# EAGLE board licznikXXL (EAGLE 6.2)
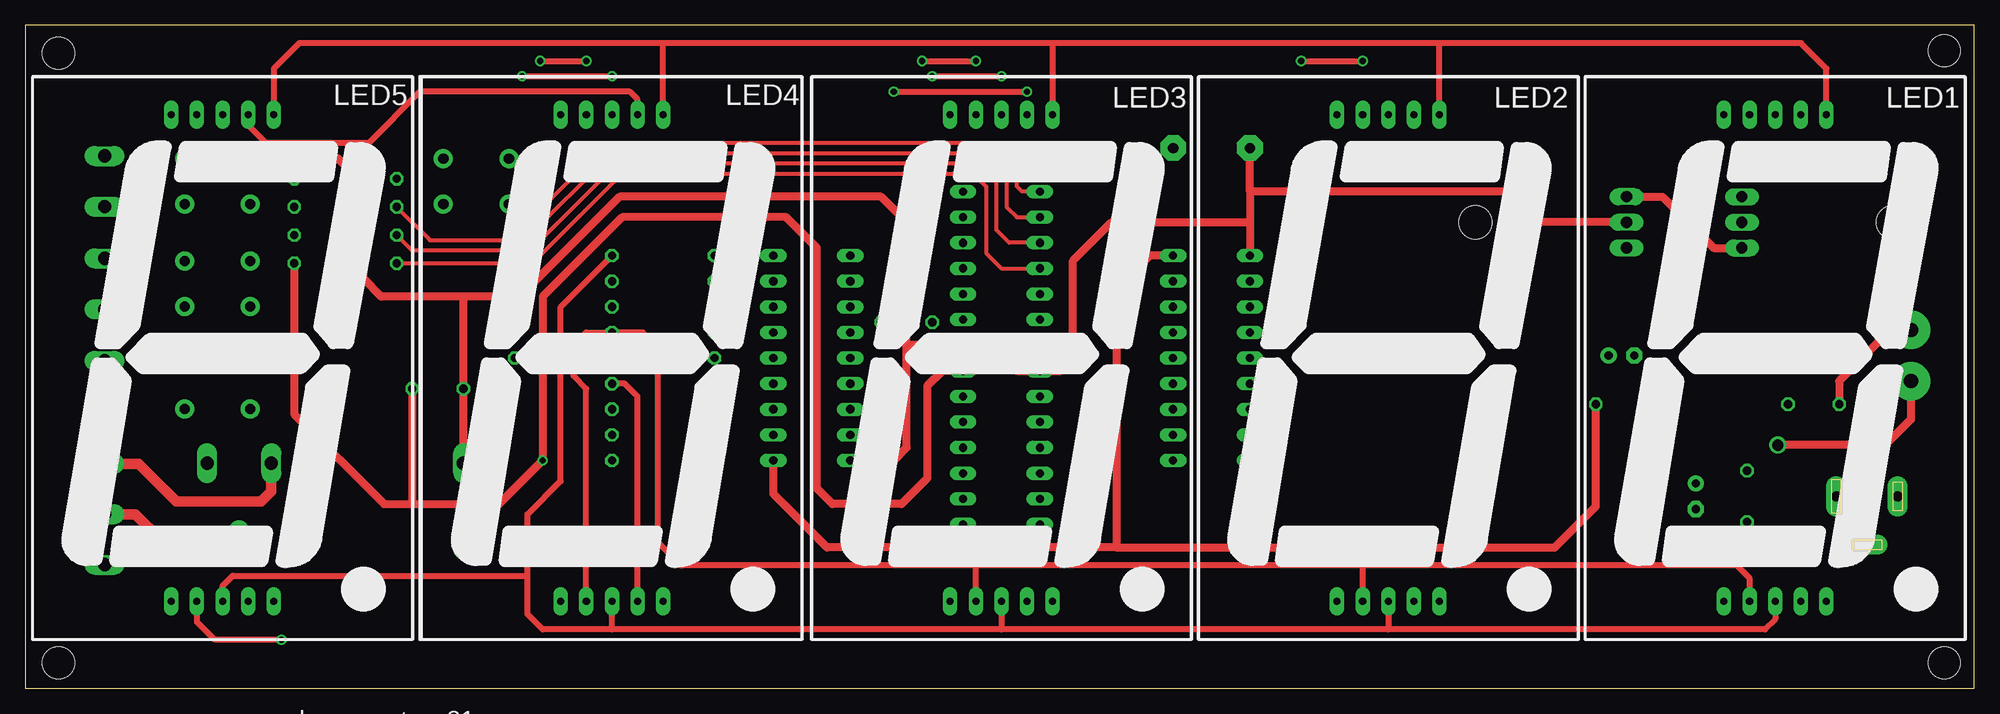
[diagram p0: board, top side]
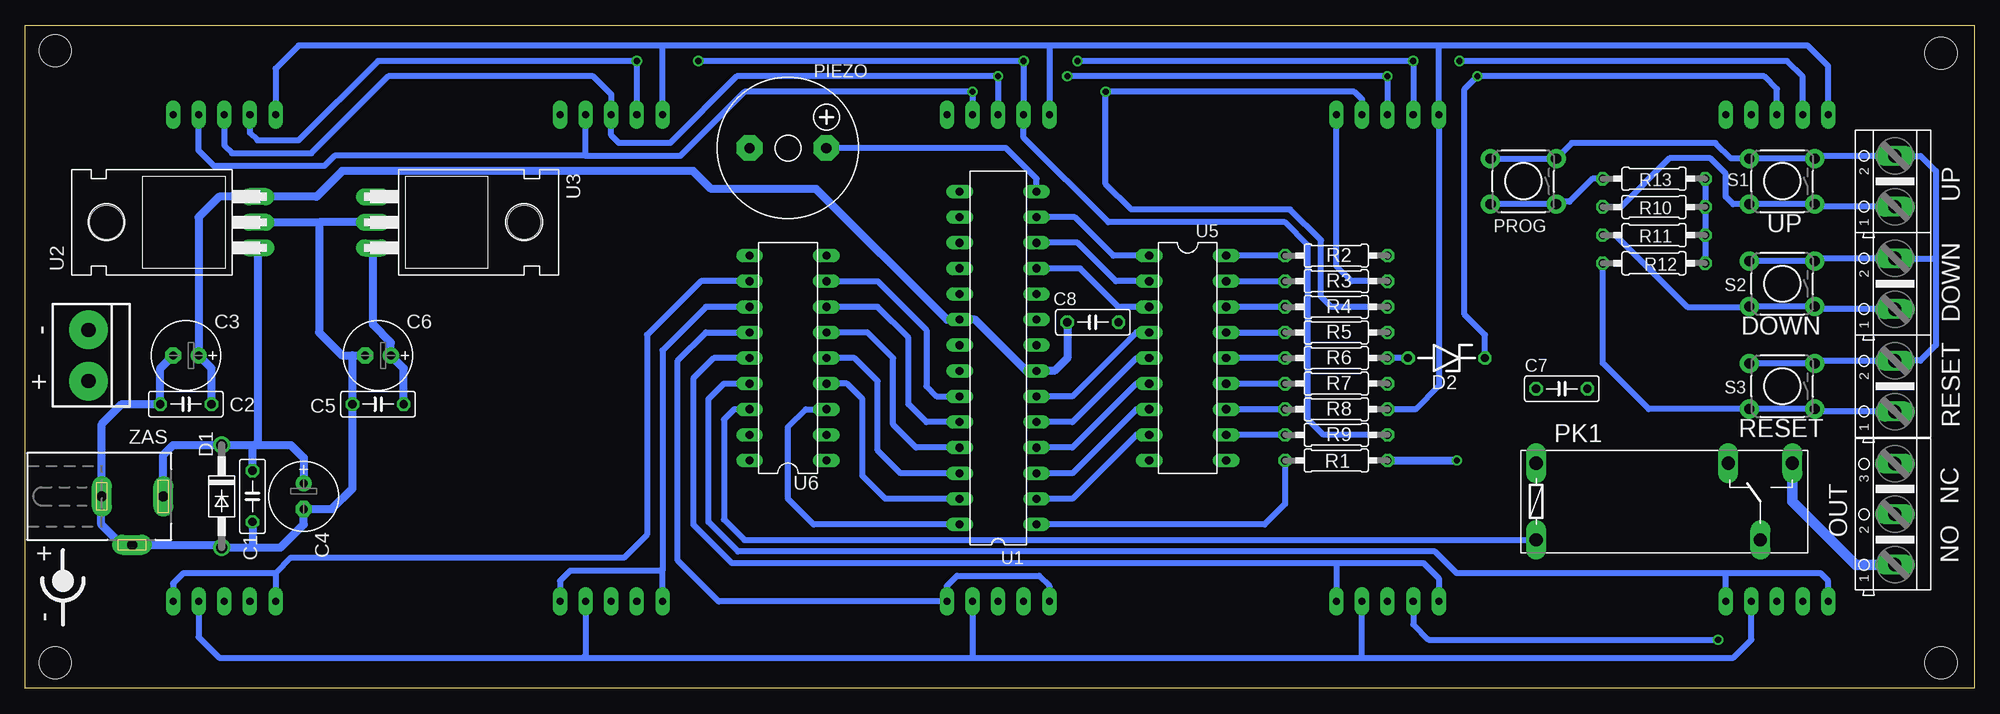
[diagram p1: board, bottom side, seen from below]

Size 193.22 x 65.78 mm. Coordinates in mm from the lower left corner, seen from the top.
Outline: 0,0 193.22,0 193.22,65.78 0,65.78 0,0
Copper layers (1*16): Top 0.035mm / dielectric 1.5mm / Bottom 0.035mm
Design rules: minimum track width 10mil, minimum drill 24mil, track to track 8mil, track to pad 8mil, pad to pad 8mil, via to via 8mil, smd to smd 8mil, copper to edge 40mil, drill to drill 8mil, minimum pad ring 10mil, minimum via ring 8mil, stop-mask expansion 4mil, vias tented up to drill 0mil, thermal gap 10mil
Holes 3.2 mm at 3.3,62.99 3.3,2.54 190.25,2.54 190.25,63.25

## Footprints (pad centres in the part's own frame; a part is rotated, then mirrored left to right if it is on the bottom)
C050-025X075 = drill 0.813 octagon: 1 -2.54,0; 2 2.54,0
E2,5-7 = drill 0.813 pad 1.6: + -1.27,0 | drill 0.813 pad 1.6 octagon: - 1.27,0
DO41-10 = drill 1.118: A 5.08,0; C -5.08,0
ZDIO-7.5 = drill 0.813 octagon: A 3.81,0; C -3.81,0
AK500/2 = drill 1.321 long: 1 -2.515,0; 2 2.515,0
SA18-11 = drill 0.7 pad 1.422 long: 1 -5.08,-24.13; 2 -2.54,-24.13; 3 0,-24.13; 4 2.54,-24.13; 5 5.08,-24.13; 6 -5.08,24.13; 7 -2.54,24.13; 8 0,24.13; 9 2.54,24.13; 10 5.08,24.13
AK500/3 = drill 1.321 long: 1 -5.004,0; 2 0,0; 3 5.004,0
F/CM12P = drill 1.016 pad 2.54 octagon: + 3.81,0; - -3.81,0
G6RW = drill 1.321 long: 1 -12.7,-3.81; 2 -12.7,3.81; O 6.35,3.81; P 9.525,-3.81; S 12.7,3.81
TACTILE-PTH = drill 1.016 pad 1.88: 1 -3.251,2.261; 2 3.251,2.261; 3 -3.251,-2.261; 4 3.251,-2.261
0207/10 = drill 0.813 octagon: 1 -5.08,0; 2 5.08,0
DIL28-3 = drill 0.813 long: 1 -16.51,-3.81; 2 -13.97,-3.81; 3 -11.43,-3.81; 4 -8.89,-3.81; 5 -6.35,-3.81; 6 -3.81,-3.81; 7 -1.27,-3.81; 8 1.27,-3.81; 9 3.81,-3.81; 10 6.35,-3.81; 11 8.89,-3.81; 12 11.43,-3.81; 13 13.97,-3.81; 14 16.51,-3.81; 15 16.51,3.81; 16 13.97,3.81; 17 11.43,3.81; 18 8.89,3.81; 19 6.35,3.81; 20 3.81,3.81; 21 1.27,3.81; 22 -1.27,3.81; 23 -3.81,3.81; 24 -6.35,3.81; 25 -8.89,3.81; 26 -11.43,3.81; 27 -13.97,3.81; 28 -16.51,3.81
TO220H = drill 1.118 long: 1 -2.54,-10.16; 2 0,-10.16; 3 2.54,-10.16 | hole 3.302: 0,4.826
DIL18 = drill 0.813 long: 1 -10.16,-3.81; 2 -7.62,-3.81; 3 -5.08,-3.81; 4 -2.54,-3.81; 5 0,-3.81; 6 2.54,-3.81; 7 5.08,-3.81; 8 7.62,-3.81; 9 10.16,-3.81; 10 10.16,3.81; 11 7.62,3.81; 12 5.08,3.81; 13 2.54,3.81; 14 0,3.81; 15 -2.54,3.81; 16 -5.08,3.81; 17 -7.62,3.81; 18 -10.16,3.81
DCJ0202 = drill 1 pad 2 long: 1 0,3.1; 2 4.8,0; 3 0,-3

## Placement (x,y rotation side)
C1  100n  [C050-025X075]  170.69,19.05 90 bottom
C2  100n  [C050-025X075]  177.29,28.19 0 bottom
C3  100u  [E2,5-7]  177.29,33.02 180 bottom
C4  220u  [E2,5-7]  165.61,19.05 270 bottom
C5  100n  [C050-025X075]  158.24,28.19 0 bottom
C6  100u  [E2,5-7]  158.24,33.02 180 bottom
C7  100n  [C050-025X075]  40.89,29.72 0 bottom
C8  100n  [C050-025X075]  87.38,36.32 180 bottom
D1  1N4007  [DO41-10]  173.74,19.05 270 bottom
D2  5V1  [ZDIO-7.5]  52.32,32.77 180 bottom
DOWN  [AK500/2]  7.87,40.13 90 bottom
LED1  7-SEG_SA18-11  [SA18-11]  173.48,32.77 0 top
LED2  7-SEG_SA18-11  [SA18-11]  135.13,32.77 0 top
LED3  7-SEG_SA18-11  [SA18-11]  96.77,32.77 0 top
LED4  7-SEG_SA18-11  [SA18-11]  58.17,32.77 0 top
LED5  7-SEG_SA18-11  [SA18-11]  19.56,32.77 0 top
OUT  [AK500/3]  7.87,17.27 90 bottom
PIEZO  F/CM12P  [F/CM12P]  117.6,53.59 0 bottom
PK1  G6RW  [G6RW]  30.73,18.54 0 bottom
PROG  [TACTILE-PTH]  44.7,50.29 180 bottom
R1  10k  [0207/10]  63.25,22.61 180 bottom
R2  [0207/10]  63.25,42.93 0 bottom
R3  [0207/10]  63.25,40.39 0 bottom
R4  [0207/10]  63.25,37.85 0 bottom
R5  [0207/10]  63.25,35.31 0 bottom
R6  [0207/10]  63.25,32.77 0 bottom
R7  [0207/10]  63.25,30.23 0 bottom
R8  [0207/10]  63.25,27.69 0 bottom
R9  [0207/10]  63.25,25.15 0 bottom
R10  10k  [0207/10]  31.75,47.75 180 bottom
R11  10k  [0207/10]  31.75,44.96 180 bottom
R12  10k  [0207/10]  31.75,42.16 180 bottom
R13  10k  [0207/10]  31.75,50.55 180 bottom
RESET  [AK500/2]  7.87,29.97 90 bottom
S1  [TACTILE-PTH]  19.05,50.29 180 bottom
S2  [TACTILE-PTH]  19.05,40.13 180 bottom
S3  [TACTILE-PTH]  19.05,29.97 180 bottom
U1  MEGA8-P  [DIL28-3]  96.77,32.77 90 bottom
U2  7805  [TO220H]  180.34,46.23 90 bottom
U3  7812  [TO220H]  148.59,46.23 270 bottom
U5  ULN2803  [DIL18]  77.98,32.77 270 bottom
U6  UDN2983A  [DIL18]  117.6,32.77 90 bottom
UP  [AK500/2]  7.87,50.29 90 bottom
ZAS  [DCJ0202]  182.63,19.05 270 bottom

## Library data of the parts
C1-C8 R1-R13 = rcl
D1 D2 = diode
DOWN OUT RESET UP = con-ptr500; OC_FARNELL: unknown; OC_NEWARK: unknown
LED1-LED5 = display-kingbright; OC_FARNELL: unknown; OC_NEWARK: unknown
PIEZO = buzzer; OC_FARNELL: unknown; OC_NEWARK: unknown
PK1 = relay; OC_FARNELL: unknown; OC_NEWARK: unknown
PROG S1-S3 = moja2
U1 = atmel; OC_FARNELL: unknown; OC_NEWARK: unknown
U2 U3 = linear
U5 U6 = uln-udn
ZAS = con-jack; OC_FARNELL: unknown; OC_NEWARK: unknown

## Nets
A: U1.2 U5.8
A1: U1.23 U6.8
A1`: LED1.1 LED1.5 U6.11
A2: U1.24 U6.7
A2`: LED2.1 LED2.5 U6.12
A3: U1.25 U6.6
A3`: LED3.1 LED3.5 U6.13
A4: U1.26 U6.5
A4`: LED4.1 LED4.5 U6.14
A5: U1.27 U6.4
A5`: LED5.1 LED5.5 U6.15
A`: LED1.7 LED2.7 LED3.7 LED4.7 LED5.7 R9.2
B: U1.3 U5.7
B`: LED1.6 LED2.6 LED3.6 LED4.6 LED5.6 R8.2
C: U1.4 U5.6
C`: LED1.4 LED2.4 LED3.4 LED4.4 LED5.4 R7.2
D: U1.13 U5.1
D`: LED1.3 LED2.3 LED3.3 LED4.3 LED5.3 R2.2
DOWN: DOWN.1 R11.2 S2.1 S2.2 U1.17
DP: U1.5 U5.5
DP`: D2.C LED1.8 LED2.8 LED3.8 LED4.8 LED5.8
E: U1.6 U5.4
E`: LED1.2 LED2.2 LED3.2 LED4.2 LED5.2 R5.2
F: U1.11 U5.3
F`: LED1.9 LED2.9 LED3.9 LED4.9 LED5.9 R4.2
G: U1.12 U5.2
G`: LED1.10 LED2.10 LED3.10 LED4.10 LED5.10 R3.2
N$1: OUT.2 PK1.P
N$2: R2.1 U5.18
N$3: R4.1 U5.16
N$4: D2.A R6.2
N$5: R5.1 U5.15
N$6: R6.1 U5.14
N$7: R7.1 U5.13
N$8: C1.2 C4.+ D1.C U2.1 U3.1 ZAS.1
N$9: R8.1 U5.12
N$10: R9.1 U5.11
N$11: R3.1 U5.17
N$12: PIEZO.+ U1.14
N$13: OUT.1 PK1.S
N$14: OUT.3 PK1.O
N$18: C1.1 C2.1 C3.- C4.- C5.1 C6.- C7.1 C8.1 D1.A DOWN.2 PIEZO.- PK1.2 PROG.3 PROG.4 RESET.2 S1.3 S1.4 S2.3 S2.4 S3.3 S3.4 U1.8 U1.22 U2.2 U3.2 U5.9 U6.10 UP.2 ZAS.2 ZAS.3
PROG: PROG.1 PROG.2 R13.2 U1.15
REL: U1.28 U6.3
REL`: PK1.1 U6.16
RES: R1.2 U1.1
RESET: R12.2 RESET.1 S3.1 S3.2 U1.18
UP: R10.2 S1.1 S1.2 U1.16 UP.1
V+: C5.2 C6.+ U3.3 U5.10 U6.9
VCC: C2.2 C3.+ C7.2 C8.2 R1.1 R10.1 R11.1 R12.1 R13.1 U1.7 U1.20 U2.3

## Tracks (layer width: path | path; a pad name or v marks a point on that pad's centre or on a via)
A
  Bottom 0.61: U5.8 83.06,25.15 89.41,18.8 U1.2
A1
  Bottom 0.61: U6.8 108.71,40.39 103.89,35.56 103.89,29.97 102.87,28.96 U1.23
A1`
  Bottom 0.61: U6.11 126.24,40.39 131.57,35.05 131.57,15.24 133.86,12.95 166.88,12.95 168.4,11.43 | 168.4,11.43 177.55,11.43 178.56,10.41 LED1.5 | 168.4,11.43 LED1.1
A2
  Bottom 0.61: U1.24 103.89,26.42 105.66,28.19 105.66,34.8 108.71,37.85 U6.7
A2`
  Bottom 0.61: U6.12 125.73,37.85 130.05,33.53 130.05,11.68 | LED2.1 130.05,11.68 | 130.05,11.68 139.19,11.68 140.21,10.67 LED2.5
A3
  Bottom 0.61: U1.25 104.9,23.88 107.19,26.16 107.19,32.77 109.73,35.31 U6.6
A3`
  Bottom 0.61: U6.13 125.73,35.31 128.52,32.51 128.52,12.7 124.46,8.64 LED3.5 101.85,10.16 100.84,11.18 92.71,11.18 91.69,10.16 LED3.1
A4
  Bottom 0.61: U1.26 106.43,21.34 108.71,23.62 108.71,30.48 111,32.77 U6.5
A4`
  Bottom 0.61: U6.14 124.97,32.77 127,30.73 127,16.26 123.19,12.45 63.25,12.45 | 63.25,12.45 LED4.5 | 63.25,12.45 54.61,12.45 53.09,10.92 LED4.1
A5
  Bottom 0.61: U1.27 107.95,18.8 110.24,21.08 110.24,28.7 111.76,30.23 U6.4
A5`
  Bottom 0.61: LED5.1 14.48,10.67 15.24,11.43 24.64,11.43 | 24.64,11.43 51.31,11.43 53.47,13.59 122.55,13.59 125.48,16.51 125.48,28.7 123.95,30.23 U6.15 | LED5.5 24.64,11.43
A`  (via drill 0.6)
  Top 0.61: v51.05,62.23 v55.63,62.23 | v88.9,62.23 v94.23,62.23 | v126.49,62.23 v132.59,62.23
  Bottom 0.61: LED5.7 17.02,60.71 18.54,62.23 v51.05,62.23 | v88.9,62.23 v55.63,62.23 LED4.7 | v126.49,62.23 v94.23,62.23 LED3.7 94.23,54.61 85.85,46.23 68.33,46.23 66.04,43.94 66.04,26.67 64.52,25.15 R9.2 | LED2.7 v132.59,62.23 158.24,62.23 166.12,54.36 170.18,54.36 170.94,55.12 LED1.7
B
  Bottom 0.61: U5.7 83.06,27.69 89.41,21.34 U1.3
B`
  Bottom 0.61: LED5.6 14.48,61.72 16.51,63.75 53.09,63.75 | 53.09,63.75 91.69,63.75 | 91.69,63.75 130.05,63.75 | 130.05,63.75 166.12,63.75 168.4,61.47 LED1.6 | LED2.6 130.05,63.75 | 53.09,63.75 LED4.6 53.09,29.97 55.37,27.69 R8.2 | 91.69,63.75 LED3.6
C
  Bottom 0.61: U5.6 83.06,30.23 89.41,23.88 U1.4
C`
  Top 0.61: LED4.4 60.71,28.96 59.44,30.23 R7.2
  Bottom 0.61: LED1.4 176.02,5.08 173.99,3.05 137.92,3.05 | 137.92,3.05 99.31,3.05 | 99.31,3.05 60.71,3.05 | 60.71,3.05 LED4.4 | LED3.4 99.31,3.05 | LED2.4 137.67,3.3 137.92,3.05 | 60.71,3.05 23.88,3.05 22.1,4.83 LED5.4
D
  Bottom 0.61: U5.1 85.34,42.93 89.15,46.74 U1.13
D`
  Top 0.61: LED1.3 173.48,6.86 172.47,5.84 135.13,5.84 | 135.13,5.84 96.77,5.84 | 96.77,5.84 58.17,5.84 | 58.17,5.84 LED4.3 | LED2.3 135.13,5.84 | LED3.3 96.77,5.84 | LED5.3 19.56,10.16 20.57,11.18 49.78,11.18 | 49.78,11.18 49.78,17.27 53.09,20.57 53.09,37.85 R2.2 | 58.17,5.84 51.31,5.84 49.78,7.37 49.78,11.18
DOWN
  Top 0.406: U1.17 97.54,44.2 96.27,45.47 96.27,50.29 94.49,52.07 58.67,52.07 50.04,43.43 38.35,43.43 R11.2
  Bottom 0.61: DOWN.1 15.55,37.62 S2.1 S2.2 22.33,37.85 28.45,37.85 35.56,44.96 R11.2
DP
  Bottom 0.61: U5.5 83.06,32.77 89.41,26.42 U1.5
DP`  (via drill 0.6)
  Top 0.61: v49.28,60.71 v58.17,60.71 | v89.92,60.71 v96.77,60.71
  Bottom 0.61: LED5.8 19.56,59.44 20.83,60.71 v49.28,60.71 50.55,59.44 50.55,37.08 48.51,35.05 D2.C | v89.92,60.71 v58.17,60.71 LED4.8 | LED3.8 v96.77,60.71 122.68,60.71 129.29,54.1 134.37,54.1 135.13,54.86 LED2.8 135.13,58.93 136.91,60.71 157.23,60.71 164.85,53.09 172.72,53.09 173.48,53.85 LED1.8
E
  Bottom 0.61: U5.4 83.06,35.31 89.41,28.96 U1.6
E`  (via drill 0.6)
  Top 0.61: LED4.2 55.63,29.72 54.36,30.99 54.36,34.04 55.63,35.31 R5.2 61.21,35.31 62.74,33.78 62.74,14.48 65.02,12.19 94.23,12.19 | LED1.2 170.94,10.92 169.67,12.19 132.59,12.19 | 132.59,12.19 94.23,12.19 | LED3.2 94.23,12.19 | LED2.2 132.59,12.19 | v25.4,4.83 18.8,4.83 17.02,6.6 LED5.2
  Bottom 0.61: LED4.2 55.63,6.35 54.1,4.83 v25.4,4.83
F
  Bottom 0.61: U5.3 84.84,37.85 88.65,41.66 U1.11
F`  (via drill 0.6)
  Top 0.61: v86.11,59.18 v99.31,59.18 | LED4.9 60.71,58.42 59.94,59.18 39.12,59.18 34.04,54.1 23.88,54.1 22.1,55.88 LED5.9
  Bottom 0.61: 137.67,52.83 162.56,52.83 163.58,51.82 174.5,51.82 176.02,53.34 LED1.9 | 137.67,52.83 LED2.9 | LED3.9 v99.31,59.18 121.92,59.18 128.27,52.83 137.67,52.83 | LED4.9 60.71,58.42 61.47,59.18 v86.11,59.18 86.11,50.04 83.57,47.5 67.82,47.5 64.77,44.45 64.77,38.86 63.75,37.85 R4.2
G
  Bottom 0.61: U5.2 85.09,40.39 88.9,44.2 U1.12
G`
  Top 0.61: LED1.10 178.56,61.47 176.02,64.01 140.21,64.01 | 140.21,64.01 101.85,64.01 | 101.85,64.01 63.25,64.01 | 63.25,64.01 27.18,64.01 24.64,61.47 LED5.10 | LED4.10 63.25,64.01 | LED2.10 140.21,64.01 | 101.85,64.01 LED3.10
  Bottom 0.61: R3.2 61.72,40.39 63.25,41.91 LED4.10
N$1
  Top 1.016: PK1.P 13.46,14.73 10.92,17.27 OUT.2
N$2
  Bottom 0.61: R2.1 U5.18
N$3
  Bottom 0.61: R4.1 U5.16
N$4
  Bottom 0.61: D2.A R6.2
N$5
  Bottom 0.61: U5.15 R5.1
N$6
  Bottom 0.61: R6.1 U5.14
N$7
  Bottom 0.61: U5.13 R7.1
N$8
  Top 0.813: U3.1 162.31,48.77 167.39,43.69 U2.1
  Bottom 0.813: ZAS.1 179.53,23.17 178.56,24.13 D1.C 170.69,24.13 | 170.69,24.13 170.43,24.13 | 170.43,24.13 166.88,24.13 165.61,22.86 C4.+ | C1.2 170.69,24.13 | U2.1 170.18,24.38 170.43,24.13
N$9
  Bottom 0.61: R8.1 U5.12
N$10
  Bottom 0.61: R9.1 U5.11
N$11
  Bottom 0.61: U5.17 R3.1
N$12
  Bottom 0.61: U1.14 92.96,50.55 96.01,53.59 113.54,53.59 113.79,53.34 PIEZO.+
N$13
  Bottom 1.016: OUT.1 11.76,12.27 18.03,18.54 PK1.S
N$14
  Top 1.016: OUT.3 11.25,22.28 14.99,18.54 23.37,18.54 24.38,19.56 PK1.O
N$15  (via drill 1.4 pad 3.81)
  other vias: 186.94,35.56
N$16  (via drill 1.4 pad 3.81)
  other vias: 186.94,30.48
N$17
  Top 0.813: 186.94,30.73 186.94,26.67 184.4,24.13 173.74,24.13
N$18
  Top 0.813: 187.2,35.56 184.91,35.56 179.83,30.48 C2.1 | 87.38,34.04 U1.8 95.76,34.04 98.3,31.5 U1.22 102.62,31.5 103.89,32.77 103.89,42.42 107.7,46.23 121.41,46.23 | 87.38,34.04 87.38,36.32 | 87.38,36.32 87.38,46.23 84.84,48.77 58.93,48.77 49.02,38.86 43.43,38.86 | 43.43,38.86 C7.1 PK1.2 | 43.43,38.86 35.31,38.86 33.53,40.64 33.53,50.04 30.99,52.58 22.33,52.58 S1.4 | U5.9 86.11,22.61 87.38,23.88 87.38,34.04 | 121.41,46.23 U6.10 | U3.2 150.11,46.23 147.07,49.28 121.41,49.28 | 121.41,49.28 PIEZO.- | 121.41,49.28 121.41,46.23 | C8.1 87.38,36.32
  Bottom 0.61: 3.81,42.42 3.81,51.31 5.31,52.81 UP.2 15.55,52.81 S1.3 S1.4 24.11,52.55 25.65,54.1 39.9,54.1 PROG.3 PROG.4 | 3.81,42.42 3.81,34.04 5.33,32.51 7.85,32.51 RESET.2 15.55,32.49 S3.3 S3.4 | 3.81,42.42 4.04,42.65 DOWN.2 15.55,42.65 S2.3 S2.4
  Bottom 0.813: 170.43,13.97 D1.A 174.02,14.25 ZAS.2 183.67,14.25 185.67,16.26 185.67,19 ZAS.3 185.63,26.21 183.64,28.19 C2.1 179.83,31.75 C3.- | 170.43,13.97 167.89,13.97 165.61,16.26 C4.- 162.81,17.78 160.78,19.81 C5.1 160.78,33.02 C6.- 161.8,33.02 164.08,35.31 164.08,46.23 | C1.1 170.69,14.22 170.43,13.97 | U2.2 164.08,46.23 | U3.2 164.08,46.23
PROG
  Top 0.406: U1.15 98.81,49.28 98.3,49.78 98.3,51.31 95.5,54.1 57.66,54.1 51.56,48.01 47.98,48.01 PROG.2
  Bottom 0.61: R13.2 37.85,50.55 40.13,48.26 41.22,48.26 PROG.1 PROG.2
REL
  Bottom 0.61: U1.28 115.06,16.26 117.6,18.8 117.6,25.91 115.82,27.69 U6.3
REL`
  Bottom 0.61: U6.16 122.94,27.69 123.95,26.67 123.95,16.76 121.92,14.73 PK1.1 43.18,14.73
RES
  Bottom 0.61: R1.2 68.33,18.29 70.36,16.26 U1.1
RESET
  Top 0.406: R12.2 50.29,42.16 59.18,51.05 93.98,51.05 95.25,49.78 95.25,43.18 96.77,41.66 U1.18
  Bottom 0.61: RESET.1 15.55,27.46 S3.1 S3.2 32.28,27.71 36.83,32.26 R12.2
UP
  Top 0.406: R10.2 40.13,44.45 49.53,44.45 58.17,53.09 95,53.09 97.28,50.8 97.28,47.75 98.3,46.74 U1.16
  Bottom 0.61: UP.1 15.55,47.78 S1.1 S1.2 23.9,48.03 24.64,48.77 24.64,51.05 26.16,52.58 30.23,52.58 35.05,47.75 R10.2
V+
  Top 0.813: U6.9 111.51,42.93 108.2,39.62 108.2,13.97 | 108.2,13.97 79.5,13.97 74.17,19.3 U5.10 | 108.2,13.97 151.64,13.97 155.7,18.03 C5.2
  Bottom 0.813: C5.2 155.7,31.75 C6.+ 156.97,34.29 158.75,36.07 U3.3
VCC  (via drill 0.6)
  Top 0.813: R12.1 26.67,27.18 35.56,18.29 38.35,18.29 | 38.35,18.29 46.99,18.29 v51.31,22.61 51.31,38.86 59.18,46.74 75.44,46.74 78.49,43.69 78.49,19.81 80.01,18.29 86.87,18.29 89.41,20.83 89.41,29.97 90.93,31.5 U1.7 | C7.2 38.35,18.29
  Bottom 0.61: R13.1 R10.1 R11.1 | R11.1 26.67,44.45 | R11.1 R12.1
  Bottom 0.813: R1.1 v51.31,22.61 | C2.2 174.75,31.75 C3.+ 176.02,46.74 173.99,48.77 U2.3 164.34,48.77 161.8,51.31 127,51.31 125.22,49.53 114.81,49.53 101.85,36.58 U1.20 99.06,36.58 93.98,31.5 U1.7 91.19,31.5 89.92,32.77 C8.2

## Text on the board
tNames: bez warstwy 21
bNames: UP | DOWN | - | + | RESET | NC | NO | + | -
tStop: mosi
